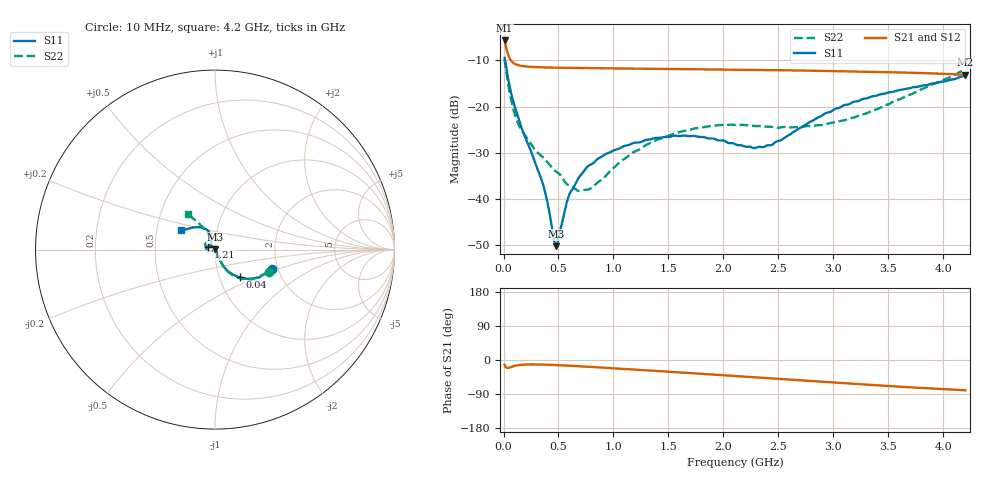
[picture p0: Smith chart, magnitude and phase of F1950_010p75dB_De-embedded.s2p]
! Integrated Device Technology
! Corporate Headquarters
! 6024 Silver Creek Valley Road
! San Jose, CA 95138  USA
! Phone:  1-408-284-8200
! Toll Free:  1-800-223-1366
! Webpage:  http://www.idt.com/
! Timing and RF Division
! 515 Groton Road, Suite 102
! Westford, MA 01886-6024
! Device:  F1950
! Description: 7-bit 0.25 dB Digital Step Attenuator
! Frequency:  150.0 -  4000.00 MHz
! Package:  4x4 mm Thin QFN Plastic Package: 24 pin
! Ports:  2 RF, 12 DC
!  Pin  1  = D0
!  Pin  2  = VDD
!  Pin  3  = Vmode
!  Pin  4  = GND
!  Pin  5  = RF1  =  Port 1
!  Pin  6  = GND
!  Pin  7  = GND
!  Pin  8  = GND
!  Pin  9  = GND
!  Pin 10  = GND
!  Pin 11  = GND
!  Pin 12  = GND
!  Pin 13  = GND
!  Pin 14  = RF2  =  Port 2
!  Pin 15  = GND
!  Pin 16  = LE
!  Pin 17  = CLK
!  Pin 18  = DATE
!  Pin 19  = D6
!  Pin 20  = D5
!  Pin 21  = D4
!  Pin 22  = D3
!  Pin 23  = D2
!  Pin 24  = D1
! State:  43
! Atten State:  10.75 dB
! Voltage:  +5.00 Volts
! Current:  Not Measured mA
! Data:  The device was measured on a the F195X evaluation board which has
!  individual transmission lines to the RF pins.  Data was collected
!  using a calibrated network analyzer.  The evaluation board was
!  de-embedded using a TRL calibration technique.
!  The reference plane is the edge of the package pin.
! Misc:  Board 2019
!  Action Tracker AT0250
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# GHz S dB R 50
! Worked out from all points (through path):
!   420 points, 10 MHz to 4.2 GHz, reference 50 ohm
!   highest |S21| = -5.69 dB at 10 MHz (marker M1); lowest = -13.1 dB at 4.2 GHz (marker M2)
!   group delay of S21, straight-line fit = 49 ps
!   lowest |S11| = -50.2 dB at 480 MHz (marker M3), VSWR 1.01, Z = 50.2 + j0.21 ohm
!   |S11| at or under -10 dB: 14.24 MHz to end of sweep
!   |S22| runs from -38.3 to -9.8 dB; largest |S21 - S12| = 0.00036
!   S11 on the Smith chart (normalised r, x): 10 MHz: 1.87, -0.45; 40 MHz: 1.25, -0.40; 1.21 GHz: 0.93, +0.03; 4.2 GHz: 0.67, +0.15
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0.01  -9.45 -18.5  -5.69 -12.6  -5.69 -12.6  -9.77 -22.7
0.04  -13.66 -48.2  -8.67 -21.1  -8.67 -21.1  -14.78 -54.3
0.09  -19.00 -62.7  -10.56 -16.5  -10.56 -16.5  -20.66 -62.9
0.15  -23.62 -65.0  -11.13 -13.1  -11.13 -13.1  -24.52 -64.8
0.36  -36.92 -47.9  -11.52 -12.1  -11.52 -12.0  -31.04 -69.3
0.4  -40.80 -40.5  -11.54 -12.4  -11.54 -12.4  -32.05 -69.4
0.46  -49.09 3.3  -11.57 -13.1  -11.57 -13.1  -33.72 -75.3
0.48  -50.24 42.8  -11.58 -13.4  -11.58 -13.4  -34.11 -78.0
0.5  -48.51 75.8  -11.59 -13.6  -11.59 -13.6  -34.46 -79.5
0.59  -39.60 116.5  -11.62 -14.9  -11.62 -15.0  -36.98 -93.0
0.71  -34.64 129.3  -11.66 -16.9  -11.66 -16.9  -38.15 -120.3
0.91  -30.60 142.2  -11.71 -20.3  -11.71 -20.3  -35.48 -165.1
1.21  -27.81 158.6  -11.79 -25.6  -11.79 -25.6  -29.57 172.5
1.41  -26.77 167.3  -11.84 -29.2  -11.84 -29.2  -27.07 165.3
1.73  -26.36 175.3  -11.92 -35.1  -11.92 -35.1  -24.79 157.1
2.11  -28.19 167.2  -12.02 -42.3  -12.02 -42.3  -24.00 147.1
2.28  -29.01 149.9  -12.07 -45.5  -12.07 -45.5  -24.21 141.4
2.43  -28.37 131.6  -12.12 -48.2  -12.12 -48.3  -24.39 136.0
2.81  -23.08 106.8  -12.24 -55.6  -12.24 -55.6  -24.26 119.5
3.1  -19.67 108.9  -12.35 -61.1  -12.35 -61.2  -22.97 113.8
3.51  -16.91 120.6  -12.55 -68.7  -12.55 -68.8  -19.42 114.9
4.2  -13.28 150.3  -13.12 -79.9  -13.12 -80.0  -11.96 127.3
